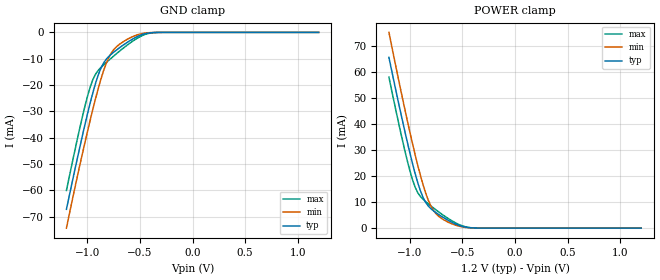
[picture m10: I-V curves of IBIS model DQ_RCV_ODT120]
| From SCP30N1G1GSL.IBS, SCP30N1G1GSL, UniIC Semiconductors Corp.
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|   Model DQ_RCV_ODT120
[Model] DQ_RCV_ODT120
Model_type Input
Vinl =  0.500V
Vinh =  0.700V
C_comp   1.373pF   1.353pF   1.403pF
[Model Spec]
Vinh   0.700V   0.670V   0.750V
Vinl   0.500V   0.470V   0.550V
[Add Submodel]
|  Submodel_name   Mode
DQ_ODT120   Non-Driving
[Temperature Range]   25.000   85.000   -40.000
[Voltage Range]   1.200V   1.140V   1.300V
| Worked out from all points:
|   GND clamp passes 1 mA (typ) near -0.49 V on its own axis
|   POWER clamp passes 1 mA (typ) near -0.53 V on its own axis
[GND_clamp]
|Voltage   I(typ)   I(min)   I(max)
-1.2V     -67.26mA   -74.42mA   -60.1mA
-1.05V    -39.62mA   -46.47mA   -32.4mA
-1V       -31.05mA   -37.77mA   -24.37mA
-950mV    -23.16mA   -29.46mA   -18.1mA
-925mV    -19.62mA   -25.5mA    -16.02mA
-875mV    -13.89mA   -18.21mA   -13.48mA
-825mV    -10.4mA    -12.16mA   -11.61mA
-775mV    -8.365mA   -7.964mA   -9.852mA
-700mV    -6.001mA   -4.671mA   -7.319mA
-525mV    -1.587mA   -933.3uA   -2.208mA
-375mV    -90.13uA   -49.22uA   -132.9uA
1.2V      0A         0A         0A
[POWER_clamp]
|Voltage   I(typ)   I(min)   I(max)
-1.2V     65.51mA    75.11mA    57.91mA
-1.05V    37.38mA    45.87mA    29.99mA
-1V       28.74mA    36.73mA    21.95mA
-950mV    20.85mA    28.08mA    15.65mA
-925mV    17.34mA    24.01mA    13.56mA
-875mV    11.74mA    16.61mA    11.06mA
-825mV    8.457mA    10.65mA    9.317mA
-775mV    6.603mA    6.7mA      7.708mA
-725mV    5.177mA    4.492mA    6.178mA
-550mV    1.336mA    943.1uA    1.707mA
-400mV    85.95uA    67.55uA    91.19uA
1.2V      0A         0A         0A
